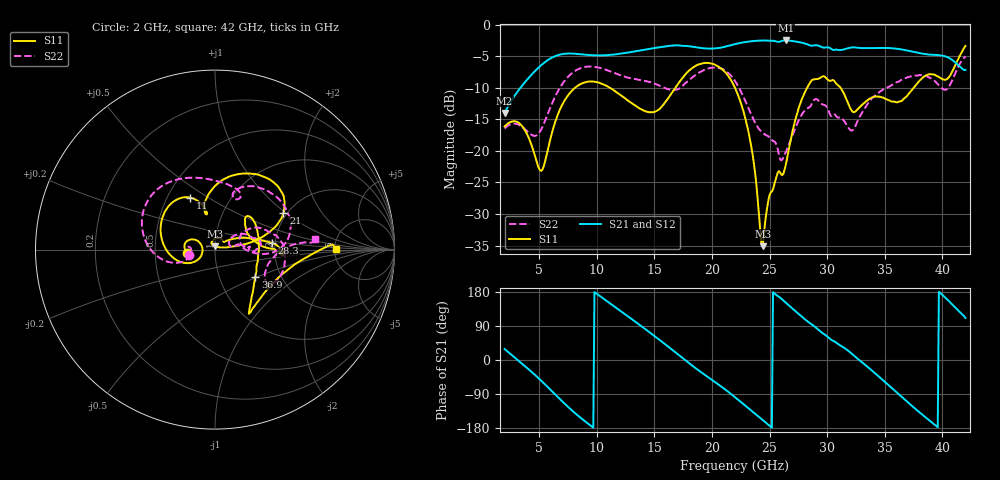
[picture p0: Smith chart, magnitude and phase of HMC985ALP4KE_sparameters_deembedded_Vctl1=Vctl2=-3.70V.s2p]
!s2p File: Measurements: S11, S21, S12, S22
# GHz S dB R 50.0
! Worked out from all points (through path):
!   401 points, 2 GHz to 42 GHz, reference 50 ohm
!   highest |S21| = -2.52 dB at 26.4 GHz (marker M1); lowest = -14.0 dB at 2 GHz (marker M2)
!   lowest |S11| = -35.1 dB at 24.4 GHz (marker M3), VSWR 1.04, Z = 50.1 + j1.76 ohm
!   |S11| at or under -10 dB: start of sweep to 8.114 GHz; 22 GHz to 28.26 GHz (6.262 GHz wide, 24.9 % of centre); 31.16 GHz to 37.51 GHz (6.351 GHz wide, 18.5 % of centre)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
!   |S22| runs from -21.5 to -5.0 dB; largest |S21 - S12| = 0.00072
!   S11 on the Smith chart (normalised r, x): 2 GHz: 0.73, -0.03; 11 GHz: 0.65, +0.42; 21 GHz: 1.91, +0.96; 28.3 GHz: 1.93, +0.15; 36.9 GHz: 1.48, -0.48; 42 GHz: 5.17, +0.11
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2  -16.13 -173.4  -14.01 29.0  -14.01 29.0  -16.45 -168.5
3.5  -16.04 160.9  -9.72 -9.4  -9.72 -9.4  -16.15 174.6
5.2  -23.16 -175.5  -6.40 -55.3  -6.40 -55.3  -16.53 -164.2
6.8  -13.46 -162.3  -4.76 -103.2  -4.76 -103.2  -10.01 -172.1
8.7  -9.33 149.5  -4.72 -155.0  -4.72 -155.1  -6.83 150.3
11  -9.86 115.5  -4.83 152.8  -4.83 152.8  -7.30 112.6
13.4  -12.90 103.0  -4.22 99.9  -4.22 99.9  -8.65 78.6
15.4  -13.44 105.2  -3.61 54.2  -3.61 54.2  -9.63 64.2
17.9  -7.48 77.1  -3.41 -5.7  -3.41 -5.7  -8.96 70.0
21  -7.28 28.3  -3.57 -74.4  -3.57 -74.4  -7.12 16.7
22  -9.99 17.7  -3.10 -98.1  -3.11 -98.1  -8.93 0.5
23.3  -18.18 9.9  -2.67 -130.5  -2.67 -130.5  -13.80 -4.1
24.4  -35.08 85.3  -2.52 -158.2  -2.53 -158.3  -17.16 9.8
25  -26.99 115.8  -2.56 -173.6  -2.56 -173.6  -17.84 12.6
26.4  -22.26 38.1  -2.52 151.5  -2.52 151.5  -20.22 32.7
28.3  -9.87 6.4  -3.15 101.7  -3.15 101.7  -13.27 18.0
28.7  -8.77 0.5  -3.36 93.2  -3.36 93.2  -12.43 15.3
32.4  -13.83 30.4  -3.62 9.6  -3.62 9.6  -16.25 26.4
35.4  -12.01 14.8  -3.73 -68.4  -3.72 -68.4  -9.81 17.0
36.9  -11.37 -33.9  -4.09 -108.9  -4.09 -108.9  -8.39 4.1
39.7  -8.30 -55.1  -4.84 180.0  -4.84 180.0  -9.62 -31.9
42  -3.40 0.5  -7.17 110.9  -7.18 110.9  -5.05 5.8
